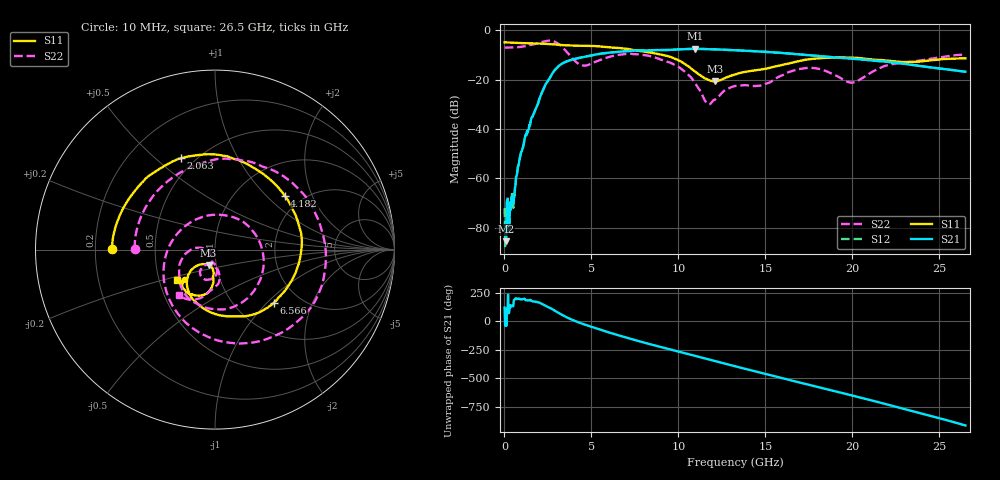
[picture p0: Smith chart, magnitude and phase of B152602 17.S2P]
!  2-Port S-parameters saved by WinCal
! VAR MeasName=S-Parameters (CALIBRATED_DATA) read from VNA (N5242A)
! VAR MeasDate=2016-1-5 16:27:47
! VAR NAME=B152602 17
! VAR FILENAME=B152602 17.S2P
! VAR DATE=2016-1-5 16:27:47
! VAR PHYS_PORTS=1,2
# Hz S DB R 50
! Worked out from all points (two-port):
!   801 points, 10 MHz to 26.5 GHz, reference 50 ohm
!   highest |S21| = -7.43 dB at 10.94 GHz (marker M1); lowest = -85.4 dB at 76.22 MHz (marker M2)
!   |S21| within 3 dB of the highest: 4.803 GHz to 18.2 GHz (13.4 GHz wide, 117 % of centre)
!   lowest |S11| = -20.7 dB at 12.1 GHz (marker M3), VSWR 1.20, Z = 45.9 - j7.93 ohm
!   |S11| at or under -10 dB: 9.14 GHz to end of sweep
!   |S22| runs from -29.9 to -4.0 dB; largest |S21 - S12| = 0.003
!   S11 on the Smith chart (normalised r, x): 10 MHz: 0.27, +0.00; 2.063 GHz: 0.42, +0.61; 4.182 GHz: 1.63, +1.29; 6.566 GHz: 1.50, -1.10; 26.5 GHz: 0.62, -0.23
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1e7  -4.84 179.6  -78.79 119.1  -72.09 24.3  -6.97 179.4
7.6225e7  -4.83 177.3  -85.42 67.6  -81.91 112.4  -6.97 175.4
4.0735e8  -4.92 165.7  -67.48 137.3  -69.02 139.8  -6.91 154.9
1.102712e9  -5.14 142.9  -46.32 -165.5  -46.38 -165.1  -6.48 111.2
2.062975e9  -5.30 110.6  -26.72 158.7  -26.71 158.7  -4.86 38.3
2.592775e9  -5.48 92.1  -19.47 117.6  -19.46 117.5  -4.07 -15.1
3.05635e9  -5.75 75.6  -14.90 77.6  -14.91 77.7  -5.20 -71.6
3.58615e9  -6.02 57.9  -12.51 33.4  -12.52 33.4  -8.68 -135.5
4.182175e9  -6.18 37.7  -11.29 -5.8  -11.30 -5.8  -13.14 150.7
4.447075e9  -6.23 28.6  -10.92 -21.0  -10.92 -20.9  -14.15 115.9
5.473562e9  -6.47 -7.4  -9.50 -73.1  -9.49 -73.0  -12.00 10.3
6.566275e9  -7.09 -41.8  -8.65 -124.2  -8.63 -124.1  -9.88 -51.3
8.851038e9  -9.56 -101.7  -7.94 139.3  -7.90 139.3  -11.43 -136.9
1.093712e10  -16.52 -139.3  -7.43 56.9  -7.43 56.9  -21.16 172.7
1.16656e10  -19.87 -127.0  -7.56 27.4  -7.54 27.5  -29.58 -155.9
1.209606e10  -20.66 -112.5  -7.66 10.7  -7.67 10.6  -28.05 -118.1
1.3255e10  -17.84 -93.4  -7.98 -34.6  -7.96 -34.7  -22.50 -105.4
1.504308e10  -15.49 -92.9  -8.68 -103.4  -8.67 -103.6  -21.57 -89.8
1.769208e10  -11.50 -106.3  -10.14 155.5  -10.10 155.6  -15.17 -110.9
2.000995e10  -11.06 -127.8  -11.42 68.3  -11.43 68.2  -21.12 -102.7
2.209604e10  -12.28 -137.3  -12.76 -13.0  -12.71 -13.3  -13.97 -87.3
2.65e10  -11.29 -141.6  -16.73 166.9  -16.72 166.7  -9.78 -128.8
